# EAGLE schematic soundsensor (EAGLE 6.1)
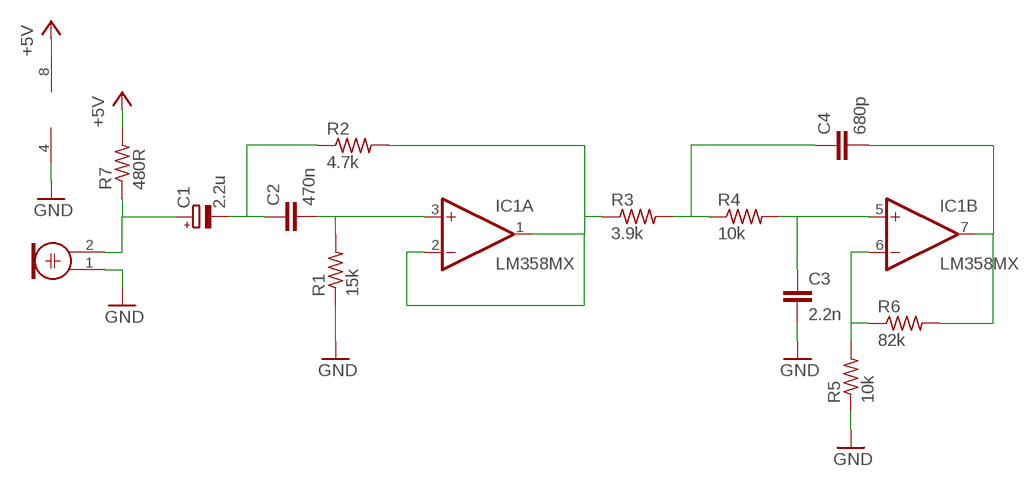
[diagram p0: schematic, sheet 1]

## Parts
C1  2.2u  CPOL-EU140CLH-1010  [140CLH-1010]
C2  470n  C-EUC1206  [C1206]
C3  2.2n  C-EUC1206  [C1206]
C4  680p  C-EUC1206  [C1206]
IC1  LM358MX  [SO08]
M1  ELECTRET_MICROPHON-WM-61A  [WM-61A]
R1  15k  R-US_R1206  [R1206]
R2  4.7k  R-US_R1206  [R1206]
R3  3.9k  R-US_R1206  [R1206]
R4  10k  R-US_R1206  [R1206]
R5  10k  R-US_R1206  [R1206]
R6  82k  R-US_R1206  [R1206]
R7  480R  R-US_R1206  [R1206]

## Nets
+5V: IC1.8(P:V+) R7.2
GND: C3.2 IC1.4(P:V-) M1.1 R1.1 R5.1
N$1: C1.- C2.1 R2.1
N$2: C2.2 IC1.3(A:+IN) R1.2
N$3: IC1.1(A:OUT) IC1.2(A:-IN) R2.2 R3.1
N$4: C4.1 R3.2 R4.1
N$5: C3.1 IC1.5(B:+IN) R4.2
N$6: IC1.6(B:-IN) R5.2 R6.1
N$7: C4.2 IC1.7(B:OUT) R6.2
N$8: C1.+ M1.2 R7.1

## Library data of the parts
C1 = resistor:CPOL-EU: POLARIZED CAPACITOR, European symbol
C2-C4 = resistor:C-EU: CAPACITOR, European symbol
IC1 = linear:LM358: OP AMP also LM158; LM258; LM2904 Source: http://cache.national.com/ds/LM/LM158.pdf
M1 = microphon:ELECTRET_MICROPHON-: Electret Condenser Microphone
R1-R7 = rcl:R-US_: RESISTOR, American symbol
